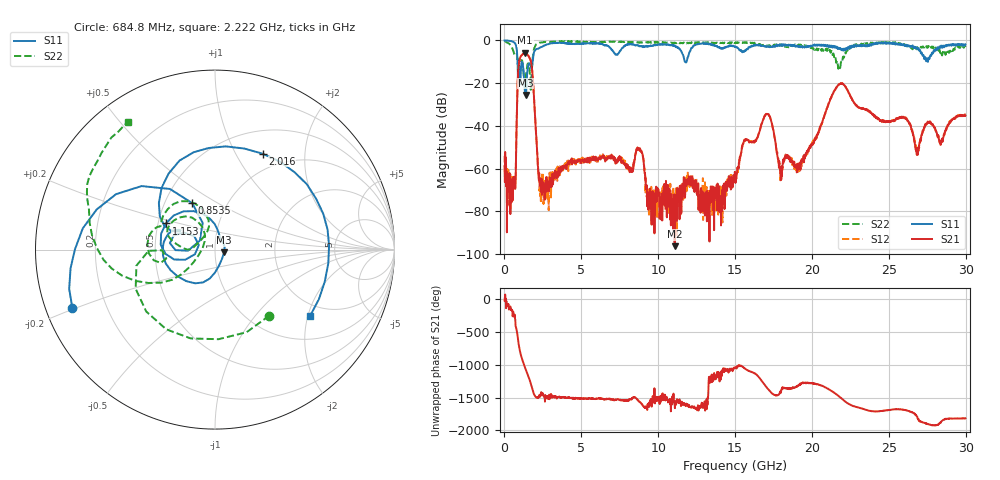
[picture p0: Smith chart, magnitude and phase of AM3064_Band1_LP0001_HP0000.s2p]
# Hz S DB R 50.0
!freq dBS11 angS11 dBS21 angS21 dBS12 angS12 dBS22 angS22
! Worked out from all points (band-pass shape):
!   1600 points, 10 MHz to 29.98 GHz, reference 50 ohm
!   highest |S21| = -5.77 dB at 1.341 GHz (marker M1); lowest = -96.4 dB at 11.07 GHz (marker M2)
!   |S21| within 3 dB of the highest: 994.3 MHz to 1.671 GHz (676.9 MHz wide, 50.8 % of centre)
!   lowest |S11| = -25.5 dB at 1.397 GHz (marker M3), VSWR 1.11, Z = 55.4 - j1.56 ohm
!   |S11| at or under -10 dB: 848.8 MHz to 1.829 GHz (980.4 MHz wide, 73.2 % of centre); 11.74 GHz to 11.84 GHz (99.99 MHz wide, 0.848 % of centre); 27.5436 GHz to 27.54467 GHz (1.07 MHz wide, 0.00389 % of centre)
!   |S22| runs from -23.1 to -0.2 dB; largest |S21 - S12| = 0.0059
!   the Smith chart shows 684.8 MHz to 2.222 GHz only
!   S11 on the Smith chart (normalised r, x): 684.8 MHz: 0.08, -0.20; 853.5 MHz: 0.69, +0.39; 1.153 GHz: 0.55, +0.18; 2.016 GHz: 0.78, +1.30; 2.222 GHz: 1.64, -2.07
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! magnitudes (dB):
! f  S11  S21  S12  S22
! 10 MHz  0.0  -58.8  -54.0  -0.2
! 684.8 MHz  -1.3  -69.2  -66.5  -6.4
! 853.5 MHz  -10.8  -20.4  -20.4  -10.6
! 1.153 GHz  -10.2  -6.8  -6.7  -9.6
! 1.341 GHz  -24.2  -5.8  -5.7  -19.6
! 1.397 GHz  -25.5  -5.9  -5.9  -16.3
! 1.734 GHz  -12.8  -10.4  -10.3  -20.2
! 2.016 GHz  -4.5  -38.4  -38.6  -2.4
! 2.222 GHz  -3.8  -64.3  -63.1  -1.3
! 5.015 GHz  -1.4  -56.0  -55.6  -0.7
! 8.763 GHz  -2.8  -50.7  -50.7  -1.1
! 9.419 GHz  -2.8  -78.8  -78.3  -0.9
! 10 GHz  -2.0  -69.6  -72.0  -0.9
! 11.07 GHz  -2.4  -96.4  -82.7  -1.0
! 15 GHz  -2.9  -64.1  -63.5  -1.3
! 17.05 GHz  -2.9  -34.4  -34.2  -2.8
! 17.99 GHz  -2.4  -65.4  -64.6  -2.4
! 19.99 GHz  -2.8  -48.8  -48.7  -3.4
! 21.85 GHz  -3.6  -20.2  -20.2  -12.4
! 25 GHz  -1.0  -38.3  -38.0  -1.1
! 26.85 GHz  -4.2  -51.3  -52.0  -3.2
! 29.98 GHz  -1.8  -35.3  -35.0  -3.1
